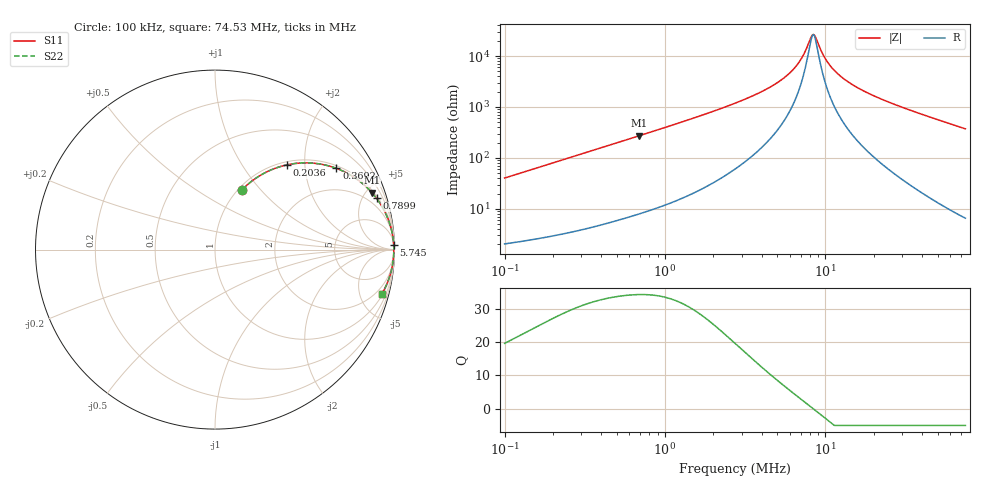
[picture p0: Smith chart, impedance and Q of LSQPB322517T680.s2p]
! LSQPB322517T680  S-PARAMETER MODEL  ( General Type )
! Model Generated by TAIYO YUDEN Corporation (http://www.ty-top.com)
! Version 2.0
! TAIYO YUDEN Control No. 100810NG22EB-FKC
! Copyright(c) 2009 TAIYO YUDEN CO.,LTD. All Rights Reserved.
! Product Description (link to TY-COMPAS)
! https://ds.yuden.co.jp/TYCOMPAS/or/detail?pn=LSQPB322517T680K&u=M
! Products Name : Inductors
! Characteristics :
!  Inductance : 68 uH , SRF(min) : 6.0 MHz , DC Resistance(max) : 1.68 Ohm
!  Rated Current : Saturation :330 mA , Temp Rise : 300 mA (40 degC)
!  Case Size : 3.2 x 2.5 / 0.126 x 0.098 [mm/inch] , Thickness : 1.7 / 0.068 [mm/inch]
!  (Conditions: Temperature = 25 degC , DC Bias Current/Voltage = 0A / 0V)
! External Node Assignments :
!  1  o---GGG---o  2
! GND o---------o GND
! Frequency Range : 0.1MHz  -  74.526194MHz  [ 402 STEP ]
# MHz S RI R 50
! Freq[MHz].  S11 Real  S11 Imag  S21 Real  S21 Imag  S12 Real  S12 Imag  S22 Real  S22 Imag
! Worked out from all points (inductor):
!   401 points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, 100 kHz to 74.53 MHz, reference 50 ohm
!   read as one part in series: L = 63.7 uH near 103.4 kHz
!   highest Q = 34.3 at 692.1 kHz (marker M1), where L = 62.8 uH
!   self-resonance near 8.265 MHz
!   S11 on the Smith chart (normalised r, x): 100 kHz: 1.04, +0.80; 203.6 kHz: 1.06, +1.62; 369.2 kHz: 1.09, +2.92; 789.9 kHz: 1.18, +6.24; 5.745 MHz: 14, +82; 74.53 MHz: 1.13, -7.46
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0.1  0.1516 0.3341  0.8484 -0.3341  0.8484 -0.3341  0.1516 0.3341
0.139192  0.2465 0.4099  0.7535 -0.4099  0.7535 -0.4099  0.2465 0.4099
0.203598  0.4007 0.4721  0.5993 -0.4721  0.5993 -0.4721  0.4007 0.4721
0.302769  0.588 0.4763  0.412 -0.4763  0.412 -0.4763  0.588 0.4763
0.369216  0.6764 0.4526  0.3236 -0.4526  0.3236 -0.4526  0.6764 0.4526
0.692071  0.8749 0.3166  0.1251 -0.3166  0.1251 -0.3166  0.8749 0.3166
0.789944  0.9002 0.2855  0.0998 -0.2855  0.0998 -0.2855  0.9002 0.2855
0.916692  0.923 0.2522  0.077 -0.2522  0.077 -0.2522  0.923 0.2522
2.729949  0.9888 0.0829  0.0112 -0.0829  0.0112 -0.0829  0.9888 0.0829
4.266142  0.9941 0.0443  0.00589 -0.0443  0.00589 -0.0443  0.9941 0.0443
5.744989  0.9956 0.0236  0.00437 -0.0236  0.00437 -0.0236  0.9956 0.0236
6.890928  0.9961 0.0121  0.00392 -0.0121  0.00392 -0.0121  0.9961 0.0121
7.362085  0.9962 0.00804  0.00382 -0.00804  0.00382 -0.00804  0.9962 0.00804
8.265445  0.9963 0.000986  0.00375 -0.000986  0.00375 -0.000986  0.9963 0.000986
8.403244  0.9963 -1.87e-05  0.00374 1.87e-05  0.00374 1.87e-05  0.9963 -1.87e-05
8.685774  0.9963 -0.00203  0.00374 0.00203  0.00374 0.00203  0.9963 -0.00203
9.591647  0.9962 -0.00808  0.0038 0.00808  0.0038 0.00808  0.9962 -0.00808
10.4183  0.9961 -0.0132  0.0039 0.0132  0.0039 0.0132  0.9961 -0.0132
12.2915  0.9957 -0.0237  0.00429 0.0237  0.00429 0.0237  0.9957 -0.0237
16.28088  0.9944 -0.0431  0.0056 0.0431  0.0056 0.0431  0.9944 -0.0431
25.02522  0.9898 -0.0798  0.0102 0.0798  0.0102 0.0798  0.9898 -0.0798
74.52619  0.9291 -0.2479  0.0709 0.2479  0.0709 0.2479  0.9291 -0.2479
